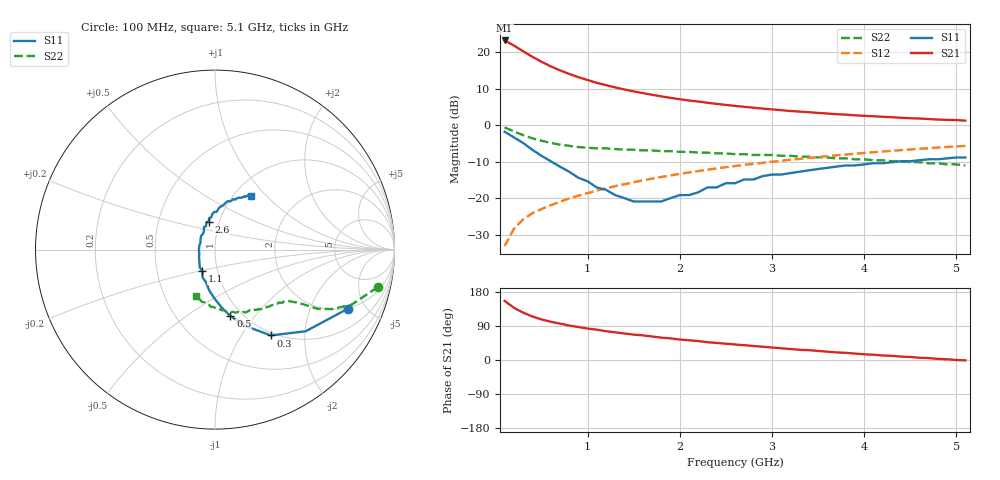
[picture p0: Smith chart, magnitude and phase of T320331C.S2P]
!AT-32033
!S PARAMETERS at Vce=1V  Ic=5mA.  LAST UPDATED 01-05-95
# ghz s ma r 50
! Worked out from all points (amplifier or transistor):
!   51 points, 100 MHz to 5.1 GHz, reference 50 ohm
!   highest |S21| = 23.2 dB at 100 MHz (marker M1)
!   |S21| within 3 dB of that: start of sweep to 303.1 MHz
!   unconditionally stable (mu >= 1): 1.257 GHz to 2.944 GHz; 3.07 GHz to 3.13 GHz
!   at 900 MHz: K = 0.95, MSG = 16.2 dB, |S12| = -19.3 dB
!   at 2.6 GHz: K = 1.02, MAG = 7.3 dB, |S12| = -11.2 dB
!   at 5.1 GHz: K = 0.95, MSG = 3.5 dB, |S12| = -5.7 dB
!   S11 on the Smith chart (normalised r, x): 100 MHz: 1.95, -3.74; 300 MHz: 0.96, -1.36; 500 MHz: 0.88, -0.76; 1.1 GHz: 0.85, -0.21; 2.6 GHz: 0.89, +0.28; 5.1 GHz: 1.20, +0.82
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0.1  0.81 -24.0  14.4 156.0  0.022 78.0  0.93 -13.0
0.2  0.68 -42.0  12.29 138.0  0.038 70.0  0.82 -22.0
0.3  0.57 -57.0  10.25 125.0  0.051 65.0  0.73 -27.0
0.4  0.46 -68.0  8.62 115.0  0.062 64.0  0.66 -30.0
0.5  0.38 -77.0  7.36 107.0  0.071 63.0  0.61 -31.0
0.6  0.32 -84.0  6.37 101.0  0.08 63.0  0.57 -32.0
0.7  0.27 -91.0  5.62 96.0  0.089 63.0  0.54 -33.0
0.8  0.23 -98.0  5.02 91.0  0.099 63.0  0.52 -34.0
0.9  0.19 -105.0  4.53 87.0  0.108 63.0  0.5 -35.0
1  0.17 -114.0  4.14 83.0  0.117 62.0  0.49 -36.0
1.1  0.14 -120.0  3.79 80.0  0.127 62.0  0.48 -37.0
1.2  0.13 -131.0  3.52 76.0  0.136 62.0  0.48 -38.0
1.4  0.1 -153.0  3.07 70.0  0.155 61.0  0.46 -40.0
1.5  0.09 -167.0  2.89 67.0  0.165 61.0  0.46 -41.0
1.8  0.09 154.0  2.47 59.0  0.195 59.0  0.44 -45.0
2  0.11 134.0  2.26 54.0  0.215 57.0  0.43 -48.0
2.3  0.14 116.0  2.02 47.0  0.245 54.0  0.42 -52.0
2.6  0.16 103.0  1.83 41.0  0.275 52.0  0.4 -57.0
3.2  0.22 86.0  1.56 29.0  0.335 46.0  0.38 -68.0
3.5  0.25 80.0  1.47 24.0  0.365 43.0  0.36 -74.0
4.3  0.31 67.0  1.28 11.0  0.444 33.0  0.32 -91.0
5.1  0.36 56.0  1.15 -1.0  0.519 24.0  0.28 -112.0
